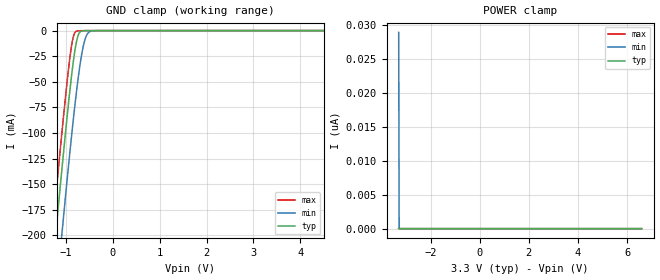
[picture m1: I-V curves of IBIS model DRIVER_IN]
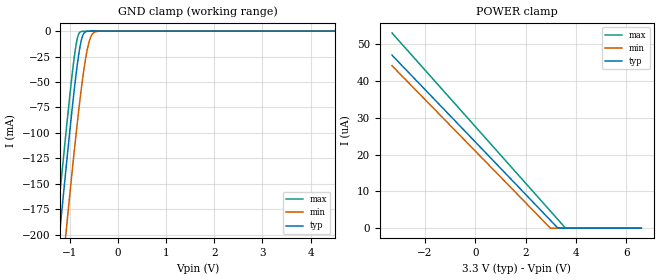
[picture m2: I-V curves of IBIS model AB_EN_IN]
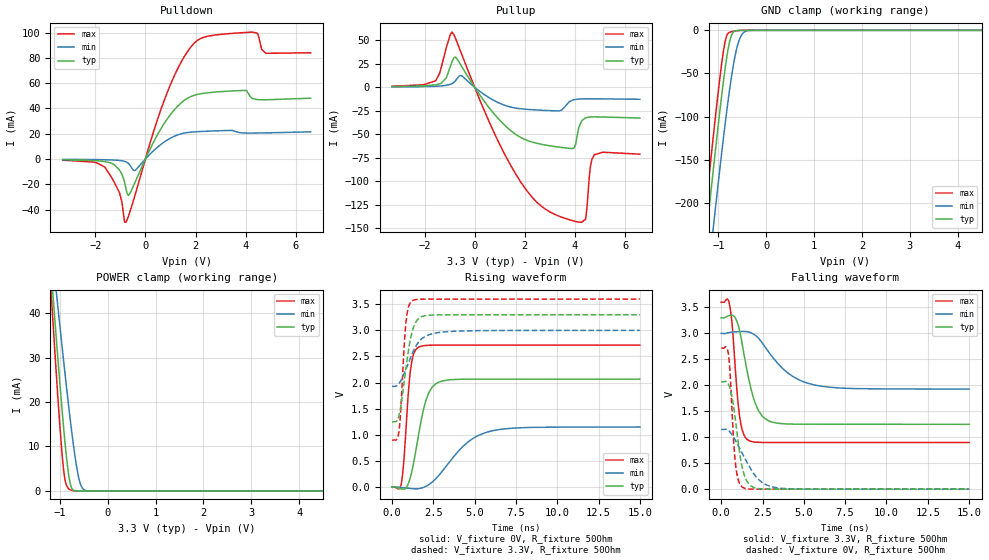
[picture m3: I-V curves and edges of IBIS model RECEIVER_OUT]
| Texas Instruments Incorporated
| CAN Transceiver Optimized for highly loaded networks
| Marketing part#   Voltage Range   Package-type   #pins/pkg drawing
| SN65HVD233D   3.0V - 3.6V   SOIC   8-pin D
| SN65HVD234D   3.0V - 3.6V   SOIC   8-pin D
| SN65HVD235D   3.0V - 3.6V   SOIC   8-pin D
[IBIS Ver]   4.0
[File name]   hvd233.ibs
[File Rev]   2.0
[Date]   10/02/2013
[Source]   Model built from TISPICED simulations at:
   Texas Instruments Incorporated.
   Analog-eLab, HPA
   12500 TI Blvd
   Dallas, TX -75243
   For Support e-mail: elab_ibis@list.ti.com
[Notes]   Revision History
   Rev 2.0: 10/02/2013
   - All new models for all pins.
   - Pullup non-monotonic on CANH and CANL buffers. This is due to short circuit current limiting
   circuit that protects against violating IOS current spec.
   - Combined pullup for RECEIVER_OUT expected and normal for this buffer.
   Rev 1.0: 05/29/2008
   - Initial model not matched to silicon
   - ccomp values are based on PVT settings:
   MIN: Low Voltage, High Temperature, Weak Process
   TYP: Nominal Voltage, Nominal Temperature, Nominal Process
   MAX: High Voltage, Low Temperature, Fast Process
   - User may change ccomp in the order of number values as
   per end simulator used
   - C_comp although listed in numberical order of value are obtained from varying PVT conditions.
   For PVT conditions for eachspecific value, refer to the buffer description under repective [Model].
   IBIS model user is responsible for using appropriate C_comp to simulate for Signal Integrity.
   - FAULT model not used on device HVD254
[Disclaimer] This model is designed as an aid for customers of Texas Instruments.
 TI and its licensors and suppliers make no warranties, either expressed
 or implied, with respect to this  model, including the warranties of
 merchantability or fitness for a particular purpose.
 The model is provided solely on an "as is" basis. The entire risk as to
 its quality and performance is with the customer.
[Copyright] (C)Copyright 2013 Texas Instruments Incorporated.
   All rights reserved.
|   Component HVD233D
[Component]   HVD233D
[Manufacturer]  Texas Instruments Incorporated
[Package]   |8-pin SOIC D package
|   typ   min   max
R_pkg   0.077174   0.00230   0.11690
L_pkg   2.321345nH   1.36253nH   2.80112nH
C_pkg   0.398513pF   0.31326pF   0.46592pF
[Pin] signal_name   model_name   R_pin   L_pin   C_pin
1   D   DRIVER_IN   0.11215   2.70023n   0.38408p
2   GND   GND   0.03900   2.09764n   0.46592p
3   VCC   POWER   0.02513   1.85198n   0.46577p
4   R   RECEIVER_OUT   0.11876   2.80112n   0.38992p
5   LBK   AB_EN_IN   0.00230   1.36253n   0.31326p
6   CANL   CANL   0.11690   2.72346n   0.40067p
7   CANH   CANH   0.09586   2.40528n   0.38694p
8   RS   NC   0.10729   2.62852n   0.38154p
[Diff_pin]   inv_pin   vdiff   tdelay_typ   tdelay_min   tdelay_max
| The CANH and CANL are Diff_pins
7   6   0.5V   0 0 0
|   Component HVD234D
[Component]   HVD234D
[Manufacturer]  Texas Instruments Incorporated
[Package]   |8-pin SOIC D package
|   typ   min   max
R_pkg   0.077174   0.00230   0.11690
L_pkg   2.321345nH   1.36253nH   2.80112nH
C_pkg   0.398513pF   0.31326pF   0.46592pF
[Pin] signal_name   model_name   R_pin   L_pin   C_pin
1   D   DRIVER_IN   0.11215   2.70023n   0.38408p
2   GND   GND   0.03900   2.09764n   0.46592p
3   VCC   POWER   0.02513   1.85198n   0.46577p
4   R   RECEIVER_OUT   0.11876   2.80112n   0.38992p
5   EN   AB_EN_IN   0.00230   1.36253n   0.31326p
6   CANL   CANL   0.11690   2.72346n   0.40067p
7   CANH   CANH   0.09586   2.40528n   0.38694p
8   RS   NC   0.10729   2.62852n   0.38154p
[Diff_pin]   inv_pin   vdiff   tdelay_typ   tdelay_min   tdelay_max
| The CANH and CANL are Diff_pins
7   6   0.5V   0 0 0
|   Component HVD235D
[Component]   HVD235D
[Manufacturer]  Texas Instruments Incorporated
[Package]   |8-pin SOIC D package
|   typ   min   max
R_pkg   0.077174   0.00230   0.11690
L_pkg   2.321345nH   1.36253nH   2.80112nH
C_pkg   0.398513pF   0.31326pF   0.46592pF
[Pin] signal_name   model_name   R_pin   L_pin   C_pin
1   D   DRIVER_IN   0.11215   2.70023n   0.38408p
2   GND   GND   0.03900   2.09764n   0.46592p
3   VCC   POWER   0.02513   1.85198n   0.46577p
4   R   RECEIVER_OUT   0.11876   2.80112n   0.38992p
5   AB   AB_EN_IN   0.00230   1.36253n   0.31326p
6   CANL   CANL   0.11690   2.72346n   0.40067p
7   CANH   CANH   0.09586   2.40528n   0.38694p
8   RS   NC   0.10729   2.62852n   0.38154p
[Diff_pin]   inv_pin   vdiff   tdelay_typ   tdelay_min   tdelay_max
| The CANH and CANL are Diff_pins
7   6   0.5V   0 0 0
[Model Selector] CANH
CANH_0   CANH RS = 0
CANH_10k   CANH RS = 10k Ohm
CANH_100k   CANH RS = 100k Ohm
[Model Selector] CANL
CANL_0   CANL RS = 0
CANL_10k   CANL RS = 10k Ohm
CANL_100k   CANL RS = 100k Ohm
| Models and submodels in the file (9): DRIVER_IN (Input), AB_EN_IN (Input), RECEIVER_OUT (3-state), CANH_0 (Open_source), CANH_10k (Open_source), CANH_100k (Open_source), CANL_0 (Open_drain), CANL_10k (Open_drain), CANL_100k (Open_drain)
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|   Driver Input Model
[Model]   DRIVER_IN
Model_type   Input
Vinl = .4
Vinh = 2.4
|   typ   min   max
|   (nom PVT)   (fast PVT)   (slow PVT)
C_comp   8.113p   7.681p   8.572p
[Voltage Range]   3.3   3   3.6
[Temperature Range]   27   150   -40
[Power Clamp Reference]   3.3   3   3.6
[GND Clamp Reference]   -0   -0   -0
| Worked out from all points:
|   GND clamp passes 1 mA (typ) near -0.69 V on its own axis
[GND Clamp]
|   Voltage   I(typ)   I(min)   I(max)
-3.3V     -1.207A    -1.293A    -1.154A
-1.815V   -490.3mA   -559.7mA   -449.2mA
-1.231V   -205.3mA   -269.5mA   -168.7mA
-1.201V   -190.9mA   -254.9mA   -154.5mA
-1.073V   -129.4mA   -192.4mA   -93.87mA
-894.3mV  -50.06mA   -109.6mA   -19.4mA
-844.8mV  -31.36mA   -88.17mA   -6.452mA
-775.5mV  -11.12mA   -60.19mA   -583.8uA
-716.1mV  -2.452mA   -39.01mA   -175.8uA
-617.1mV  -106.6uA   -12.8mA    -76.14uA
-458.7mV  -23.49uA   -505.4uA   -27.58uA
6.59V     0A         0A         0A
[POWER Clamp]
|   Voltage   I(typ)   I(min)   I(max)
-3.3V     43.4pA     28.88nA    46.42pA
-3.28V    0A         0A         0A
-3.27V    0A         0A         0A
6.59V     0A         0A         0A
|   AB/EN/LBK Input Model
[Model]   AB_EN_IN
Model_type   Input
Vinl = .4
Vinh = 2.4
|   typ   min   max
|   (nom PVT)   (fast PVT)   (slow PVT)
C_comp   8.113p   7.681p   8.572p
[Voltage Range]   3.3   3   3.6
[Temperature Range]   27   150   -40
[Power Clamp Reference]   3.3   3   3.6
[GND Clamp Reference]   -0   -0   -0
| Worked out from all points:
|   GND clamp passes 1 mA (typ) near -0.69 V on its own axis
[GND Clamp]
|   Voltage   I(typ)   I(min)   I(max)
-3.3V     -1.207A    -1.293A    -1.154A
-1.815V   -490.3mA   -559.7mA   -449.2mA
-1.231V   -205.3mA   -269.5mA   -168.7mA
-1.201V   -190.9mA   -254.9mA   -154.5mA
-1.073V   -129.4mA   -192.4mA   -93.86mA
-894.3mV  -50.06mA   -109.6mA   -19.4mA
-844.8mV  -31.35mA   -88.17mA   -6.442mA
-775.5mV  -11.12mA   -60.18mA   -569.9uA
-716.1mV  -2.445mA   -39.01mA   -160.7uA
-617.1mV  -90.91uA   -12.79mA   -58.72uA
-458.7mV  -3.55uA    -497.4uA   -4.84uA
6.59V     0A         0A         0A
[POWER Clamp]
|   Voltage   I(typ)   I(min)   I(max)
-3.3V     47.01uA    44.15uA    53.03uA
2.977V    2.185uA    13.1nA     4.689uA
3.274V    52.5nA     0A         2.397uA
3.58V     0A         0A         22.68nA
6.59V     0A         0A         0A
|   Receiver Output MODEL
[Model]   RECEIVER_OUT
Model_type   3-state
Polarity   Non-Inverting
Vref = 3.3
Cref = 15pF
Rref = 50
|   typ   min   max
|   (nom PVT)   (fast PVT)   (slow PVT)
C_comp   11.349p   9.406fp   11.706p
|C_comp (Hi state)   11.425p   11.022p   11.851p
|C_comp (Low state)   11.349p   9.406fp   11.706p
[Voltage Range]   3.3   3   3.6
[Temperature Range]   27   150   -40
[Pullup Reference]   3.3   3   3.6
[Pulldown Reference]   -0   -0   -0
[Power Clamp Reference]   3.3   3   3.6
[GND Clamp Reference]   -0   -0   -0
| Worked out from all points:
|   slope of the pulldown table from 0 to 0.495 V, typ, clamps not added: 25.2 ohm
|   slope of the pullup table from 0 to 0.495 V, typ, clamps not added: 26.2 ohm
|   GND clamp passes 1 mA (typ) near -0.66 V on its own axis
|   POWER clamp passes 1 mA (typ) near -0.77 V on its own axis
|   falling waveform, V_fixture 3.3V, R_fixture 50Ohm: 20-80 % time 840ps typ, 1.94ns min, 408ps max; typ from 3.3 V to 1.25 V
|   rising waveform, V_fixture 0V, R_fixture 50Ohm: 20-80 % time 769ps typ, 2ns min, 368ps max; typ from 0 V to 2.07 V
|   rising waveform, V_fixture 3.3V, R_fixture 50Ohm: 20-80 % time 566ps typ, 936ps min, 297ps max; typ from 1.25 V to 3.3 V
|   falling waveform, V_fixture 0V, R_fixture 50Ohm: 20-80 % time 556ps typ, 1.24ns min, 298ps max; typ from 2.07 V to 0 V
[Pulldown]
|   Voltage   I(typ)   I(min)   I(max)
-3.3V     -581.9uA   -251.5uA   -931.3uA
-1.627V   -2.001mA   -575.5uA   -6.297mA
-1.043V   -8.466mA   -1.119mA   -26.29mA
-765.6mV  -24.3mA    -2.311mA   -49.89mA
-666.6mV  -28.75mA   -3.659mA   -44.7mA
-409.2mV  -18.23mA   -9.002mA   -28.28mA
838.2mV   30.76mA    14.62mA    50.98mA
1.987V    50.69mA    21.5mA     92.46mA
4.026V    54.18mA    20.58mA    100.2mA
4.264V    47.88mA    20.57mA    100.5mA
4.808V    46.87mA    20.68mA    83.66mA
6.59V     48.14mA    21.52mA    84.08mA
[GND Clamp]
|   Voltage   I(typ)   I(min)   I(max)
-3.3V     -1.316A    -1.377A    -1.287A
-1.36V    -294mA     -360mA     -256.4mA
-1.241V   -231.6mA   -298.2mA   -193.5mA
-1.102V   -159.8mA   -227.1mA   -121.2mA
-884.4mV  -54.99mA   -120.5mA   -20.9mA
-825mV    -31.48mA   -93.82mA   -6.353mA
-755.7mV  -11.15mA   -65.16mA   -2.089mA
-686.4mV  -2.029mA   -40.4mA    -1.129mA
-597.3mV  -138.3uA   -16.98mA   -379.9uA
-518.1mV  -14.64uA   -5.789mA   -68.95uA
-399.3mV  -222.6nA   -503.5uA   -1.15uA
6.59V     0A         0A         0A
[Pullup]
|   Voltage   I(typ)   I(min)   I(max)
-3.3V     649.1uA    369.9uA    1.049mA
-1.558V   2.637mA    1.084mA    7.008mA
-1.132V   9.879mA    2.071mA    42.13mA
-904.2mV  27.16mA    3.876mA    58.79mA
-528mV    22.58mA    12.33mA    35.93mA
1.779V    -52.55mA   -22.71mA   -98.42mA
2.779V    -61.35mA   -24.62mA   -129.1mA
3.977V    -64.32mA   -13.22mA   -142.6mA
4.422V    -32.64mA   -12.32mA   -140.6mA
4.61V     -31.71mA   -12.29mA   -86.02mA
4.778V    -31.54mA   -12.31mA   -71.85mA
6.59V     -32.8mA    -12.79mA   -71.28mA
[POWER Clamp]
|   Voltage   I(typ)   I(min)   I(max)
-3.3V     367.3mA    289.1mA    436.7mA
-1.171V   47.93mA    54.98mA    42.79mA
-1.122V   40.94mA    49.79mA    34.3mA
-1.063V   32.7mA     43.61mA    24.42mA
-963.6mV  19.52mA    33.49mA    9.585mA
-924mV    14.59mA    29.53mA    5.023mA
-864.6mV  7.9mA      23.71mA    1.335mA
-765.6mV  985uA      14.53mA    182.6uA
-607.2mV  2.803uA    3.046mA    1.522uA
-547.8mV  197.3nA    984.3uA    64.34nA
-448.8mV  0A         81.02uA    0A
6.59V     0A         0A         0A
[Ramp]
R_load = 50
|   typ   min   max
dV/dt_r   1.2402/7.68899e-10   0.689619/2.00206e-09   1.63077/3.68277e-10
dV/dt_f   1.23098/8.39617e-10   0.643396/1.93941e-09   1.62082/4.08011e-10
[Falling Waveform]
V_fixture = 3.3V
V_fixture_min = 3V
V_fixture_max = 3.6V
R_fixture = 50Ohm
C_fixture = 0F
|   Time   V(typ)   V(min)   V(max)
0s        3.3V       3V         3.6V
498.9ps   3.343V     3.016V     3.562V
656.1ps   3.351V     3.023V     3.198V
1.113ns   3.055V     3.034V     1.406V
1.381ns   2.6V       3.037V     1.043V
1.687ns   2.095V     3.024V     934.1mV
2.234ns   1.526V     2.914V     903.7mV
3.323ns   1.275V     2.459V     899.1mV
6.137ns   1.251V     1.979V     899mV
15ns      1.248V     1.928V     898.6mV
[Rising Waveform]
V_fixture = 0V
V_fixture_min = 0V
V_fixture_max = 0V
R_fixture = 50Ohm
C_fixture = 0F
|   Time   V(typ)   V(min)   V(max)
0s        -442.4pV   9.643nV    197.2nV
577.5ps   -36.01mV   -11.39mV   82.45mV
734.7ps   -39.56mV   -16.73mV   559.4mV
1.113ns   182.6mV    -27.32mV   2.218V
1.572ns   925.8mV    -32.77mV   2.672V
2.234ns   1.808V     46.18mV    2.715V
3.064ns   2.033V     310.1mV    2.718V
4.637ns   2.066V     871.1mV    2.718V
6.137ns   2.066V     1.081V     2.718V
15ns      2.067V     1.149V     2.718V
[Rising Waveform]
V_fixture = 3.3V
V_fixture_min = 3V
V_fixture_max = 3.6V
R_fixture = 50Ohm
C_fixture = 0F
|   Time   V(typ)   V(min)   V(max)
0s        1.248V     1.928V     898.6mV
429.1ps   1.376V     1.982V     1.071V
538.2ps   1.552V     2.037V     1.496V
734.7ps   2V         2.167V     2.667V
852.6ps   2.285V     2.258V     3.158V
996.5ps   2.609V     2.373V     3.443V
1.285ns   3.041V     2.595V     3.577V
1.793ns   3.262V     2.837V     3.597V
3.14ns    3.298V     2.97V      3.6V
15ns      3.3V       3V         3.6V
[Falling Waveform]
|Gnd
V_fixture = 0V
V_fixture_min = 0V
V_fixture_max = 0V
R_fixture = 50Ohm
C_fixture = 0F
|   Time   V(typ)   V(min)   V(max)
0s        2.067V     1.149V     2.718V
429.1ps   2.027V     1.133V     2.62V
538.2ps   1.939V     1.099V     2.238V
734.7ps   1.626V     1.009V     1.029V
852.6ps   1.356V     943.9mV    525.2mV
1.055ns   842mV      823.8mV    156.2mV
1.381ns   290.3mV    625.5mV    20.69mV
2.295ns   10.01mV    175.9mV    259.1uV
3.439ns   1.087mV    24.27mV    235.8uV
15ns      -442.4pV   518.3nV    197.2nV
